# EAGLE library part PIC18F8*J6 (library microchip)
PIC18F97J60 Family 64/80/100-Pin High-Performance, 1-Mbit Flash Microcontrollers with Ethernet Source: http://ww1.microchip.com/downloads/en/DeviceDoc/39762d.pdf
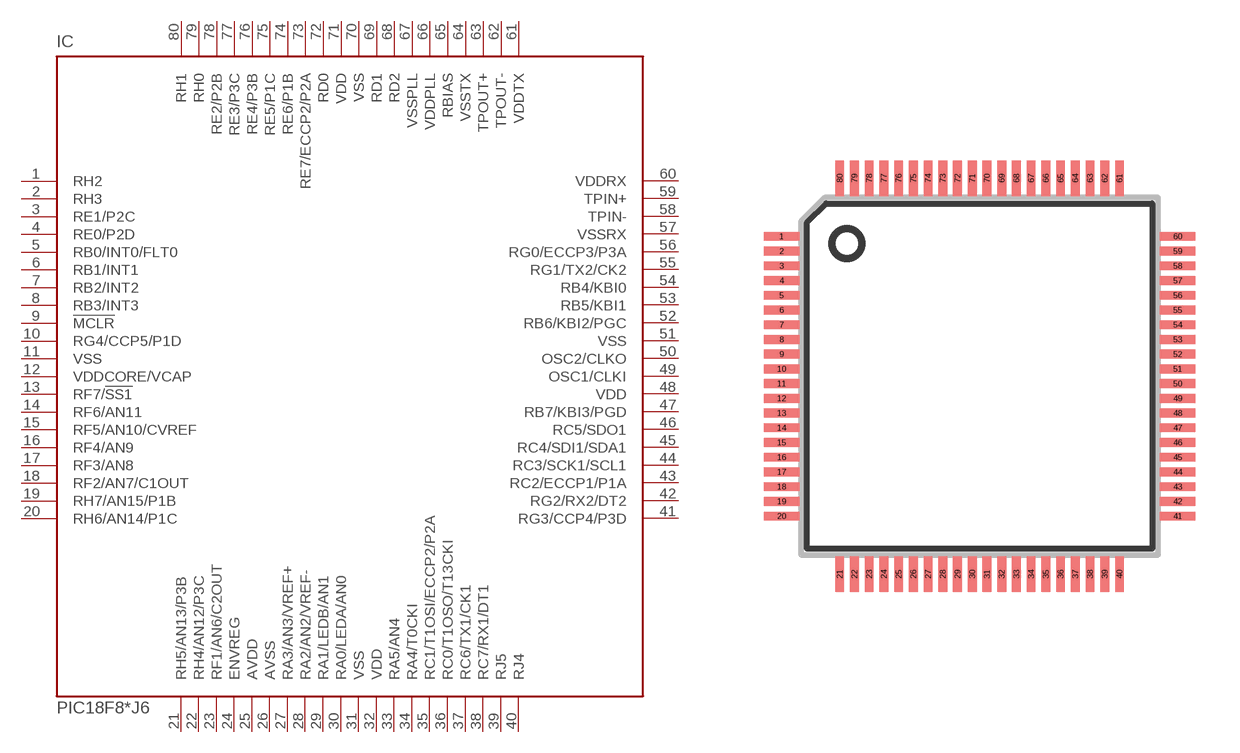
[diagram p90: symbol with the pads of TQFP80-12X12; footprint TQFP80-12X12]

Designator prefix IC

## PIC18F86J60 (MPN: PIC18F86J60-I/PT; OC_FARNELL: unknown; OC_NEWARK: 56K7306), PIC18F87J60 (MPN: PIC18F87J60-I/PT; OC_FARNELL: 1332291; OC_NEWARK: 56K7312)  [TQFP80-12X12]
1  RH2
2  RH3
3  RE1/P2C
4  RE0/P2D
5  RB0/INT0/FLT0
6  RB1/INT1
7  RB2/INT2
8  RB3/INT3
9  !MCLR  in
10  RG4/CCP5/P1D
11  VSS  pwr
12  VDDCORE/VCAP  in
13  RF7/!SS1
14  RF6/AN11
15  RF5/AN10/CVREF
16  RF4/AN9
17  RF3/AN8
18  RF2/AN7/C1OUT
19  RH7/AN15/P1B
20  RH6/AN14/P1C
21  RH5/AN13/P3B
22  RH4/AN12/P3C
23  RF1/AN6/C2OUT
24  ENVREG  in
25  AVDD  in
26  AVSS  in
27  RA3/AN3/VREF+
28  RA2/AN2/VREF-
29  RA1/LEDB/AN1
30  RA0/LEDA/AN0
31  VSS  pwr
32  VDD  pwr
33  RA5/AN4
34  RA4/T0CKI
35  RC1/T1OSI/ECCP2/P2A
36  RC0/T1OSO/T13CKI
37  RC6/TX1/CK1
38  RC7/RX1/DT1
39  RJ5
40  RJ4
41  RG3/CCP4/P3D
42  RG2/RX2/DT2
43  RC2/ECCP1/P1A
44  RC3/SCK1/SCL1
45  RC4/SDI1/SDA1
46  RC5/SDO1
47  RB7/KBI3/PGD
48  VDD  pwr
49  OSC1/CLKI  in
50  OSC2/CLKO  out
51  VSS  pwr
52  RB6/KBI2/PGC
53  RB5/KBI1
54  RB4/KBI0
55  RG1/TX2/CK2
56  RG0/ECCP3/P3A
57  VSSRX  in
58  TPIN-  in
59  TPIN+  in
60  VDDRX  in
61  VDDTX  in
62  TPOUT-  out
63  TPOUT+  out
64  VSSTX  in
65  RBIAS  in
66  VDDPLL  in
67  VSSPLL  in
68  RD2
69  RD1
70  VSS  pwr
71  VDD  pwr
72  RD0
73  RE7/ECCP2/P2A
74  RE6/P1B
75  RE5/P1C
76  RE4/P3B
77  RE3/P3C
78  RE2/P2B
79  RH0
80  RH1

## PIC18F86J65 (MPN: PIC18F86J65-I/PT; OC_FARNELL: 1564571; OC_NEWARK: 95M7065)  [TQFP80-12X12]
Pads as for TQFP80-12X12

## Footprint TQFP80-12X12 (pad centres in mm)
TQFP80 12x12x1 mm Body Source: http://www.microchip.com/ .. 39663c.pdf
smd 1.2 x 0.3: 1 -6.725,4.75; 2 -6.725,4.25; 3 -6.725,3.75; 4 -6.725,3.25; 5 -6.725,2.75; 6 -6.725,2.25; 7 -6.725,1.75; 8 -6.725,1.25; 9 -6.725,0.75; 10 -6.725,0.25; 11 -6.725,-0.25; 12 -6.725,-0.75; 13 -6.725,-1.25; 14 -6.725,-1.75; 15 -6.725,-2.25; 16 -6.725,-2.75; 17 -6.725,-3.25; 18 -6.725,-3.75; 19 -6.725,-4.25; 20 -6.725,-4.75; 41 6.725,-4.75; 42 6.725,-4.25; 43 6.725,-3.75; 44 6.725,-3.25; 45 6.725,-2.75; 46 6.725,-2.25; 47 6.725,-1.75; 48 6.725,-1.25; 49 6.725,-0.75; 50 6.725,-0.25; 51 6.725,0.25; 52 6.725,0.75; 53 6.725,1.25; 54 6.725,1.75; 55 6.725,2.25; 56 6.725,2.75; 57 6.725,3.25; 58 6.725,3.75; 59 6.725,4.25; 60 6.725,4.75
smd 0.3 x 1.2: 21 -4.75,-6.725; 22 -4.25,-6.725; 23 -3.75,-6.725; 24 -3.25,-6.725; 25 -2.75,-6.725; 26 -2.25,-6.725; 27 -1.75,-6.725; 28 -1.25,-6.725; 29 -0.75,-6.725; 30 -0.25,-6.725; 31 0.25,-6.725; 32 0.75,-6.725; 33 1.25,-6.725; 34 1.75,-6.725; 35 2.25,-6.725; 36 2.75,-6.725; 37 3.25,-6.725; 38 3.75,-6.725; 39 4.25,-6.725; 40 4.75,-6.725; 61 4.75,6.725; 62 4.25,6.725; 63 3.75,6.725; 64 3.25,6.725; 65 2.75,6.725; 66 2.25,6.725; 67 1.75,6.725; 68 1.25,6.725; 69 0.75,6.725; 70 0.25,6.725; 71 -0.25,6.725; 72 -0.75,6.725; 73 -1.25,6.725; 74 -1.75,6.725; 75 -2.25,6.725; 76 -2.75,6.725; 77 -3.25,6.725; 78 -3.75,6.725; 79 -4.25,6.725; 80 -4.75,6.725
